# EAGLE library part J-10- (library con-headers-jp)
HEADER JACK PINS
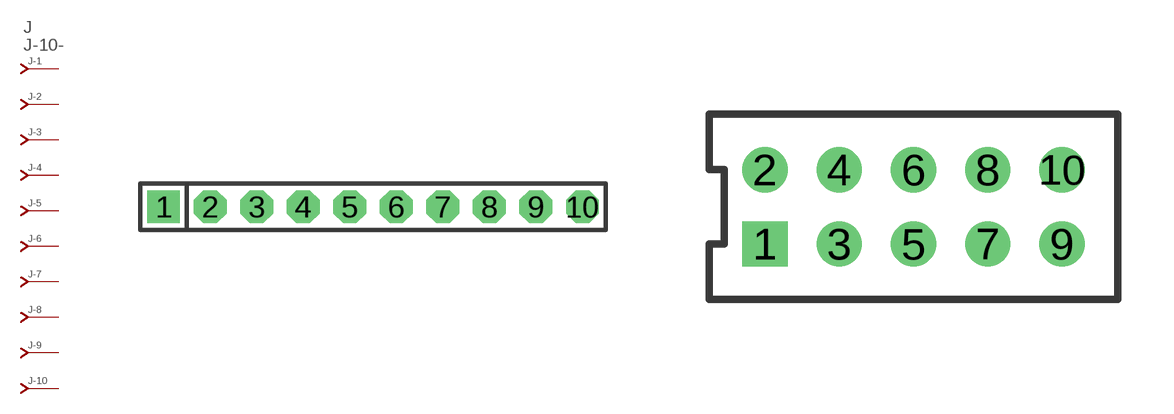
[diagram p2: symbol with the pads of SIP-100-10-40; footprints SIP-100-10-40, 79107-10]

Designator prefix J; gates -2=J-N -3=J-N -4=J-N -5=J-N -6=J-N -7=J-N -8=J-N -9=J-N -10=J-N -1=J-NV

## J-10-SIP-100-40  [SIP-100-10-40]
1  -1:J  pas
2  -2:J  pas
3  -3:J  pas
4  -4:J  pas
5  -5:J  pas
6  -6:J  pas
7  -7:J  pas
8  -8:J  pas
9  -9:J  pas
10  -10:J  pas

## J-10-79107  [79107-10]
Pads as for SIP-100-10-40

## J-10-79109  [79109-10]
Pads as for SIP-100-10-40

## J-10-87264  [87264-10]
Pads as for SIP-100-10-40

## J-10-87340  [87340-10]
Pads as for SIP-100-10-40

## J-10-87368  [87368-10]
Pads as for SIP-100-10-40

## J-10-100-2X05  [DIL-100-2X05]
Pads as for SIP-100-10-40

## J-10-100-2X05_M  [DIL-100-2X05_M]
Pads as for SIP-100-10-40

## J-10-2MM-2X05  [DIL-2MM-2X05]
Pads as for SIP-100-10-40

## J-10-2MM-2X05_M  [DIL-2MM-2X05_M]
Pads as for SIP-100-10-40

## J-10-535512  [535512-10]
Pads as for SIP-100-10-40

## J-10-SIP-100-32  [SIP-100-10-32]
Pads as for SIP-100-10-40

## J-10-SIP-100-40Y  [SIP-100-10-40Y]
Pads as for SIP-100-10-40

## J-10-SIP-100-32Y  [SIP-100-10-32Y]
Pads as for SIP-100-10-40

## J-10-71991  [71991-10]
Pads as for SIP-100-10-40

## J-10-KK-4455-B10  [KK-4455-B10]
Pads as for SIP-100-10-40

## J-10-KK-4455-A10  [KK-4455-A10]
Pads as for SIP-100-10-40

## J-10-KK-4455-C10  [KK-4455-C10]
Pads as for SIP-100-10-40

## Footprint SIP-100-10-40 (pad centres in mm)
SIP Header - 0.1", 40 mil drill
drill 1.016 pad 1.778 square: 1 -11.43,0
drill 1.016 pad 1.778 octagon: 2 -8.89,0; 3 -6.35,0; 4 -3.81,0; 5 -1.27,0; 6 1.27,0; 7 3.81,0; 8 6.35,0; 9 8.89,0; 10 11.43,0

## Footprint 79107-10 (pad centres in mm)
Molex Board-To-Board Receptacal 2.00mm (.079") Pitch Milli-Grid Header, Vertical, Through-Hole Mates with: 87759, 87762, 87758, 87760
drill 0.711 square: 1 -4,-1
drill 0.711: 2 -4,1; 3 -2,-1; 4 -2,1; 5 0,-1; 6 0,1; 7 2,-1; 8 2,1; 9 4,-1; 10 4,1

## Footprint 79109-10 (pad centres in mm)
Molex Board-to-Board Receptacal 2.00mm (.079") Pitch Milli-Grid Header, Vertical, Top/Bottom Entry Mates with: 87758, 87759, 87760, 87831, 87832, 87833
smd 1.12 x 1.83: 1 -4,-2.65; 2 -4,2.65; 3 -2,-2.65; 4 -2,2.65; 5 0,-2.65; 6 0,2.65; 7 2,-2.65; 8 2,2.65; 9 4,-2.65; 10 4,2.65
hole 0.914 at -3,0
hole 0.914 at -4,1
hole 0.914 at -4,-1
hole 0.914 at -2,-1
hole 0.914 at -2,1
hole 0.914 at 0,-1
hole 0.914 at 0,1
hole 0.914 at 3,0
hole 0.914 at 2,1
hole 0.914 at 2,-1
hole 0.914 at 4,1
hole 0.914 at 4,-1

## Footprint 87264-10 (pad centres in mm)
Molex Board-To-Board Receptacal 2.00mm (.079") Pitch Milli-Grid Header, Side Entry Mates with 2mm(.079") Mill-Grid Header
drill 0.914 square: 1 -4,-2.25
drill 0.914: 2 -4,2.25; 3 -2,-2.25; 4 -2,2.25; 5 0,-2.25; 6 0,2.25; 7 2,-2.25; 8 2,2.25; 9 4,-2.25; 10 4,2.25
